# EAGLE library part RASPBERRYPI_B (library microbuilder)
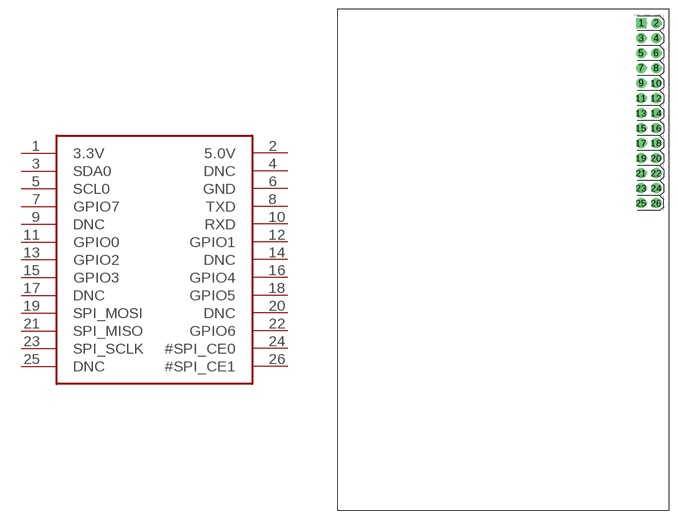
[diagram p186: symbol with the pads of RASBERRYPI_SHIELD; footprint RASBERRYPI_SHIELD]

Designator prefix -

## RASPBERRYPI_BB  [RASBERRYPI_SHIELD]
1  3.3V  sup
2  5.0V  sup
3  SDA0
4  DNC  nc
5  SCL0  out
6  GND  sup
7  GPIO7
8  TXD  out
9  DNC  nc
10  RXD  in
11  GPIO0
12  GPIO1
13  GPIO2
14  DNC  nc
15  GPIO3
16  GPIO4
17  DNC  nc
18  GPIO5
19  SPI_MOSI  out
20  DNC  nc
21  SPI_MISO  in
22  GPIO6
23  SPI_SCLK  out
24  #SPI_CE0  out
25  DNC  nc
26  #SPI_CE1  out

## Footprint RASBERRYPI_SHIELD (pad centres in mm)
drill 1 pad 1.676 square: 1 51.308,82.55
drill 1 pad 1.676: 2 53.848,82.55; 3 51.308,80.01; 4 53.848,80.01; 5 51.308,77.47; 6 53.848,77.47; 7 51.308,74.93; 8 53.848,74.93; 9 51.308,72.39; 10 53.848,72.39; 11 51.308,69.85; 12 53.848,69.85; 13 51.308,67.31; 14 53.848,67.31; 15 51.308,64.77; 16 53.848,64.77; 17 51.308,62.23; 18 53.848,62.23; 19 51.308,59.69; 20 53.848,59.69; 21 51.308,57.15; 22 53.848,57.15; 23 51.308,54.61; 24 53.848,54.61; 25 51.308,52.07; 26 53.848,52.07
